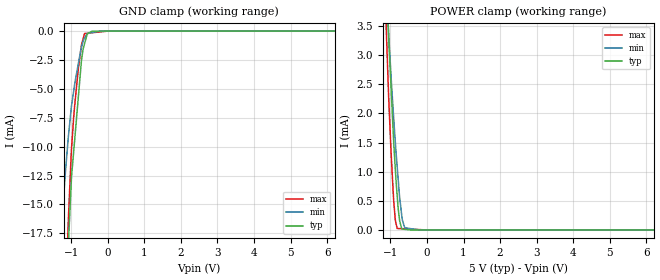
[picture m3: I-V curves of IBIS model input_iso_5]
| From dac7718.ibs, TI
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|   input_iso_5 Model
[Model]   input_iso_5
Model_type   Input
Vinl = 0.8
Vinh = 3.8
|   typ   min   max
|   (Nom PVT)   (Fast PVT)   (Slow PVT)
|C_comp from frequency method(F=50MHz)
|Average
|C_comp   3.761e-12   3.730e-12   4.269e-12
|C_comp from LC tank method(L=1nH)
|Resonant Frequency(Hz)   3.3e9   3.3e9   3.2e9
C_comp   2.328e-12   2.327e-12   2.476e-12
| Where nom  PVT is Nominal Process,  5V,  33C
|   Fast PVT is Strong Process,   5.5V,  -40C
|   Slow PVT is Weak Process,   4.5V,  113C
[Voltage Range]   5   4.5   5.5
|Ambient Temperature   25   85   -40
|Junction Temperature
[Temperature Range]   33   113   -40
[Power Clamp Reference]   5   4.5   5.5
[GND Clamp Reference]   0   0   0
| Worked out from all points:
|   GND clamp passes 1 mA (typ) near -0.62 V on its own axis
|   POWER clamp passes 1 mA (typ) near -0.86 V on its own axis
[GND Clamp]
|   Voltage   I(typ)   I(min)   I(max)
-5V       -466.2mA   -326.7mA   -519.6mA
-1.269V   -34.46mA   -17.29mA   -35.09mA
-1.14V    -23.38mA   -11.6mA    -22.08mA
-1.08V    -18.75mA   -9.263mA   -16.72mA
-994.5mV  -12.93mA   -6.584mA   -10.45mA
-907.5mV  -9.572mA   -4.693mA   -6.587mA
-803mV    -5.702mA   -2.817mA   -3.247mA
-715mV    -2.443mA   -1.373mA   -1.158mA
-632.5mV  -1.088mA   -584.3uA   -210.5uA
-560mV    -251.9uA   -230.6uA   -186.4uA
-435mV    -11.66uA   -131.8uA   -144.8uA
10V       0A         0A         0A
[POWER Clamp]
|   Voltage   I(typ)   I(min)   I(max)
-5V       81.16mA    67.53mA    96.55mA
-1.134V   4.735mA    4.484mA    3.906mA
-1.105V   4.27mA     4.12mA     3.346mA
-1.053V   3.414mA    3.45mA     2.413mA
-979mV    2.429mA    2.625mA    1.323mA
-913mV    1.574mA    1.965mA    553.5uA
-863.5mV  1.045mA    1.505mA    169.8uA
-814mV    596uA      1.096mA    25.18uA
-745mV    154.4uA    557.4uA    23.05uA
-679.5mV  22.42uA    203.8uA    21.02uA
-607.5mV  10.87uA    37.96uA    18.8uA
10V       0A         0A         0A
